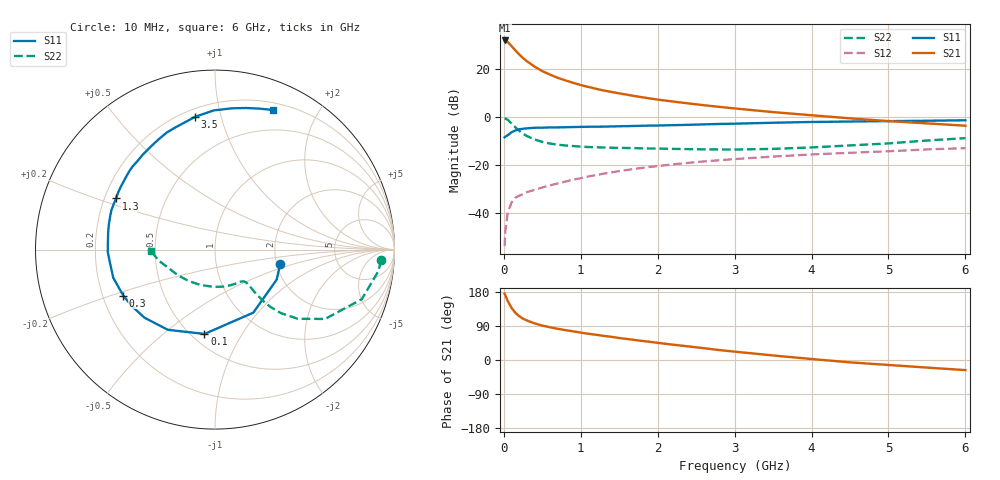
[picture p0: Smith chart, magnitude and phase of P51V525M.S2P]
! SIEMENS Small Signal Semiconductors
! BFP183
! Si NPN RF Bipolar Junction Transistor in SOT143
! VCE = 1.5 V  IC = 25 mA
! Common Emitter S-Parameters:  March  1996
# GHz  S  MA  R  50
!  f  S11  S21  S12  S22
! GHz  MAG  ANG  MAG  ANG  MAG  ANG  MAG  ANG
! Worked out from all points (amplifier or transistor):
!   36 points, 10 MHz to 6 GHz, reference 50 ohm
!   highest |S21| = 31.8 dB at 10 MHz (marker M1)
!   |S21| within 3 dB of that: start of sweep to 118.4 MHz
!   unconditionally stable (mu >= 1): 543.3 MHz to end of sweep
!   at 250 MHz: K = 0.64, MSG = 28.3 dB, |S12| = -32.3 dB
!   at 1.4 GHz: K = 1.26, MAG = 13.7 dB, |S12| = -23.2 dB
!   at 6 GHz: K = 1.01, MAG = 4.0 dB, |S12| = -13.1 dB
!   S11 on the Smith chart (normalised r, x): 10 MHz: 2.09, -0.40; 100 MHz: 0.58, -0.70; 300 MHz: 0.29, -0.22; 1.3 GHz: 0.25, +0.23; 3.5 GHz: 0.25, +0.83; 6 GHz: 0.27, +1.46
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0.01  0.3717 -12.8  38.81 175.0  0.002 77.9  0.9283 -3.7
0.02  0.3822 -25.9  38.65 170.2  0.0042 81.5  0.9168 -7.7
0.05  0.4111 -58.7  36.19 155.8  0.0099 74.7  0.863 -18.7
0.1  0.4735 -97.1  29.65 137.4  0.0163 58.2  0.7249 -32.2
0.15  0.5182 -120.4  24.12 124.6  0.0204 51.9  0.6011 -39.9
0.2  0.546 -135.9  19.83 115.5  0.0226 49.7  0.5089 -44.0
0.25  0.5602 -145.7  16.61 108.9  0.0243 48.1  0.4427 -46.0
0.3  0.5715 -153.4  14.32 104.3  0.0268 47.7  0.395 -46.8
0.4  0.5882 -164.5  11.06 96.6  0.0298 48.6  0.3345 -47.1
0.5  0.5897 -172.7  8.905 90.9  0.0335 49.6  0.298 -46.7
0.6  0.5977 -178.8  7.542 86.4  0.037 52.0  0.2756 -46.4
0.7  0.5984 175.5  6.462 82.4  0.0406 53.6  0.2604 -46.3
0.8  0.6027 171.0  5.707 78.8  0.0443 54.3  0.2512 -46.6
1.1  0.6175 159.2  4.166 69.2  0.0569 55.5  0.2332 -49.3
1.3  0.6209 152.7  3.515 63.6  0.065 55.5  0.2277 -52.1
1.7  0.641 140.2  2.694 52.9  0.0818 53.6  0.2213 -59.6
2.2  0.6654 126.9  2.068 40.4  0.1016 49.8  0.2132 -71.7
2.8  0.7054 112.4  1.602 26.2  0.1235 44.4  0.2078 -89.6
3.5  0.7481 98.5  1.246 12.0  0.1474 38.1  0.2134 -112.9
4.5  0.7928 83.2  0.924 -6.2  0.1767 28.6  0.2518 -145.6
5.5  0.8236 72.5  0.726 -20.0  0.2078 20.1  0.3186 -168.7
6  0.8415 67.6  0.648 -26.7  0.2207 15.4  0.3571 -178.7
